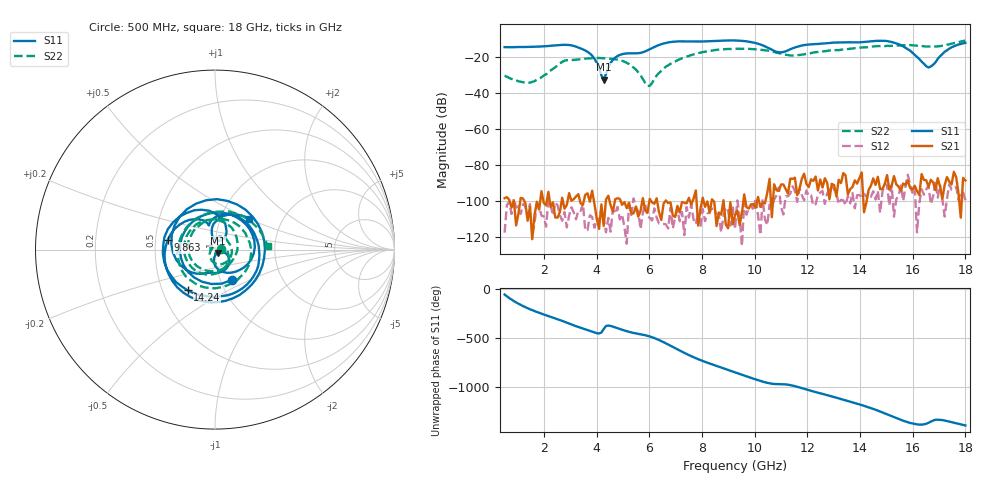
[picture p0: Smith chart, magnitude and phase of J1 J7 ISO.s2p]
!Agilent Technologies,N5230A,MY45001360,A.07.50.67
!Agilent N5230A: A.07.50.67
!Date: Tuesday, April 16, 2024 16:35:37
!Correction: S11(Full 2 Port(1,2))
!S21(Full 2 Port(1,2))
!S12(Full 2 Port(1,2))
!S22(Full 2 Port(1,2))
!S2P File: Measurements: S11, S21, S12, S22:
# Hz S  dB  R 50
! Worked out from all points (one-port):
!   201 points, 500 MHz to 18 GHz, reference 50 ohm
!   lowest |S11| = -32.4 dB at 4.263 GHz (marker M1), VSWR 1.05, Z = 51.4 - j1.95 ohm
!   |S11| at or under -10 dB: start of sweep to end of sweep
!   S11 on the Smith chart (normalised r, x): 500 MHz: 1.14, -0.40; 9.863 GHz: 0.58, +0.07; 14.24 GHz: 0.67, -0.33; 18 GHz: 1.36, +0.50
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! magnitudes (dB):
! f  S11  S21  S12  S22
! 500 MHz  -14.2  -98.3  -117.4  -30.2
! 1.462 GHz  -14.1  -103.0  -101.5  -34.0
! 2.775 GHz  -13.0  -104.1  -106.0  -21.8
! 3.475 GHz  -15.5  -101.9  -101.3  -20.9
! 3.913 GHz  -20.7  -101.6  -114.7  -20.4
! 4.263 GHz  -32.4  -113.7  -109.4  -20.4
! 4.525 GHz  -23.1  -102.1  -116.9  -20.7
! 4.787 GHz  -19.2  -98.3  -103.1  -21.2
! 5.487 GHz  -17.7  -103.0  -103.2  -26.7
! 5.925 GHz  -16.0  -106.5  -108.3  -35.8
! 6.362 GHz  -13.0  -106.0  -112.3  -28.6
! 7.588 GHz  -11.1  -101.9  -101.6  -18.7
! 9.25 GHz  -10.5  -107.8  -115.6  -15.2
! 9.863 GHz  -11.4  -101.7  -101.7  -15.3
! 11 GHz  -17.2  -90.6  -103.2  -17.8
! 12.22 GHz  -12.6  -88.7  -102.4  -17.3
! 14.24 GHz  -11.3  -100.8  -97.4  -14.4
! 15.11 GHz  -11.1  -93.6  -102.3  -13.6
! 15.9 GHz  -16.2  -92.5  -90.6  -13.1
! 16.6 GHz  -25.6  -92.0  -91.3  -13.9
! 17.39 GHz  -15.1  -89.1  -90.4  -12.7
! 18 GHz  -11.9  -88.4  -99.4  -10.6
